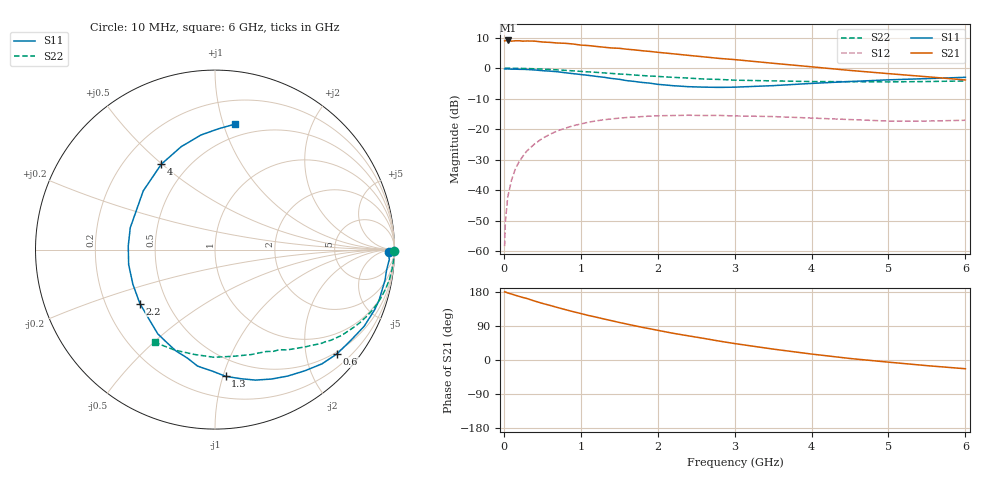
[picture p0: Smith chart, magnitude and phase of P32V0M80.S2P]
! SIEMENS Small Signal Semiconductors
! BFP181
! Si NPN RF Bipolar Junction Transistor in SOT143
! VCE = 2 V  IC = 0.8 mA
! Common Emitter S-Parameters:  March  1996
# GHz  S  MA  R  50
!  f  S11  S21  S12  S22
! GHz  MAG  ANG  MAG  ANG  MAG  ANG  MAG  ANG
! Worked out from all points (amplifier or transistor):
!   36 points, 10 MHz to 6 GHz, reference 50 ohm
!   highest |S21| = 9.1 dB at 50 MHz (marker M1)
!   |S21| within 3 dB of that: start of sweep to 1.656 GHz
!   unconditionally stable (mu >= 1): 3.308 GHz to end of sweep
!   at 250 MHz: K = 0.08, MSG = 18.8 dB, |S12| = -28.8 dB
!   at 1.4 GHz: K = 0.47, MSG = 11.6 dB, |S12| = -16.7 dB
!   at 6 GHz: K = 1.36, MAG = 3.0 dB, |S12| = -17.1 dB
!   S11 on the Smith chart (normalised r, x): 10 MHz: 52, -27; 600 MHz: 0.46, -2.64; 1.3 GHz: 0.36, -1.02; 2.2 GHz: 0.35, -0.29; 4 GHz: 0.36, +0.50; 6 GHz: 0.39, +1.09
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0.01  0.97 -0.9  2.804 179.7  0.0012 89.2  0.9979 -0.3
0.02  0.9666 -1.4  2.823 179.5  0.003 90.4  0.9977 -0.6
0.05  0.9729 -3.2  2.848 177.0  0.0076 90.5  0.9976 -1.7
0.1  0.9627 -6.8  2.776 174.1  0.0146 84.6  0.9965 -3.3
0.15  0.9625 -10.2  2.816 170.8  0.0223 83.4  0.9943 -4.8
0.2  0.9576 -13.8  2.816 167.8  0.0295 80.8  0.9923 -6.5
0.4  0.9345 -27.2  2.777 155.5  0.0571 71.7  0.9763 -12.8
0.6  0.8941 -40.5  2.648 144.1  0.0823 62.7  0.9517 -18.7
0.8  0.8403 -53.5  2.557 132.9  0.1036 54.6  0.9203 -24.2
0.9  0.8127 -60.1  2.49 127.6  0.1135 50.5  0.9031 -26.9
1.1  0.7611 -72.8  2.348 117.5  0.1297 43.5  0.8691 -31.5
1.3  0.7085 -85.2  2.206 108.3  0.1422 36.7  0.8366 -35.9
1.5  0.6563 -98.5  2.118 99.1  0.1513 31.0  0.8016 -39.8
1.8  0.5824 -117.7  1.931 86.2  0.1606 23.7  0.7561 -44.9
2.2  0.5153 -144.3  1.721 70.5  0.1671 14.8  0.7069 -51.4
2.8  0.4837 177.6  1.445 49.9  0.1677 4.6  0.6533 -60.2
3  0.4876 165.6  1.382 43.4  0.1645 1.9  0.6355 -63.3
3.5  0.5166 140.7  1.203 28.8  0.1607 -3.3  0.6183 -71.1
4  0.5619 122.2  1.052 15.7  0.1518 -6.9  0.603 -80.3
4.5  0.6036 108.2  0.918 4.0  0.1434 -9.2  0.5999 -90.6
5.5  0.6737 88.3  0.723 -14.9  0.1354 -5.1  0.6033 -112.0
6  0.708 80.9  0.64 -23.1  0.1396 -3.1  0.6163 -123.1
